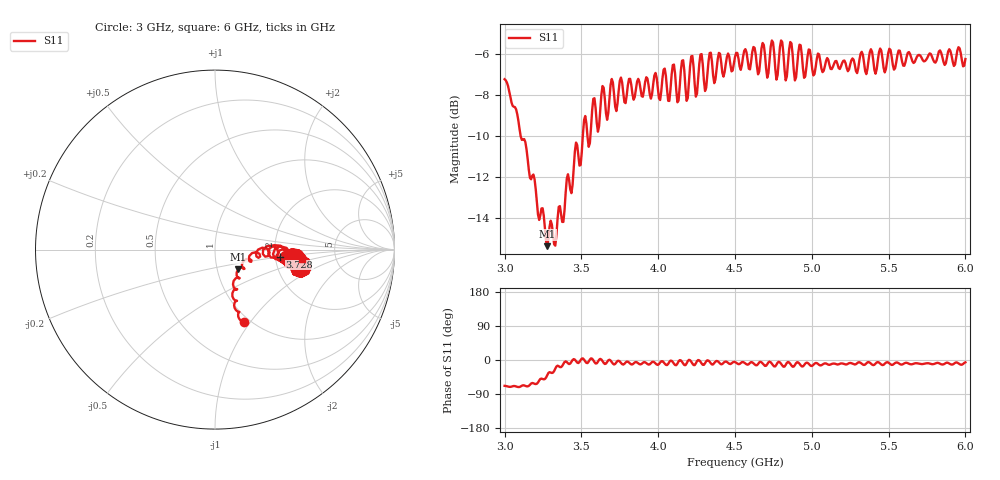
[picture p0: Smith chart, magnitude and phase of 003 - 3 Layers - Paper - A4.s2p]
!  02/07/2025  15:26:12
! Ref Plane: 0.000 mm
# MHZ S MA R  50
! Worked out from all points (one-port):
!   401 points, 3 GHz to 6 GHz, reference 50 ohm
!   lowest |S11| = -15.4 dB at 3.277 GHz (marker M1), VSWR 1.41, Z = 63.2 - j14.2 ohm
!   |S11| at or under -10 dB: 3.104 GHz to 3.509 GHz (404.8 MHz wide, 12.2 % of centre); 3.539 GHz to 3.559 GHz (19.21 MHz wide, 0.541 % of centre)
!   S11 on the Smith chart (normalised r, x): 3 GHz: 0.93, -0.93; 3.728 GHz: 2.12, -0.19; 6 GHz: 2.85, -0.39
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3000  0.4354 -68.2
3150  0.2779 -69.6
3277.5  0.1699 -40.0
3375  0.1948 -15.8
3577.5  0.3898 -0.6
3727.5  0.3639 -6.2
3750  0.4315 -4.0
4095  0.4715 -5.3
4125  0.3823 -9.6
4155  0.4831 -4.6
4185  0.3855 -9.1
4215  0.4952 -4.3
4245  0.3947 -9.0
4275  0.5004 -4.5
4305  0.4074 -8.6
4500  0.4936 -5.5
4695  0.5011 -15.5
4725  0.487 -4.3
4755  0.5044 -16.9
4785  0.4835 -4.7
4815  0.5044 -17.6
4845  0.4782 -5.2
4875  0.5016 -17.6
4905  0.4718 -5.8
4935  0.4998 -16.9
5250  0.4732 -7.8
5625  0.5052 -8.4
6000  0.4879 -6.1
